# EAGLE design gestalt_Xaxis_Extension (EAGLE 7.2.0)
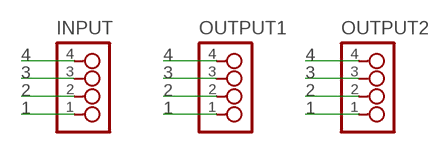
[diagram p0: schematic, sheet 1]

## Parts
INPUT  4_PIN_HEADERHEADER  [SMT_PINS_4]
OUTPUT1  4_PIN_HEADERHEADER  [SMT_PINS_4]
OUTPUT2  4_PIN_HEADERHEADER  [SMT_PINS_4]

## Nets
1: INPUT.1 OUTPUT1.1 OUTPUT2.1
2: INPUT.2 OUTPUT1.2 OUTPUT2.2
3: INPUT.3 OUTPUT1.3 OUTPUT2.3
4: INPUT.4 OUTPUT1.4 OUTPUT2.4

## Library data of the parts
INPUT OUTPUT1 OUTPUT2 = ng:4_PIN_HEADER: 4 SMT pin pads

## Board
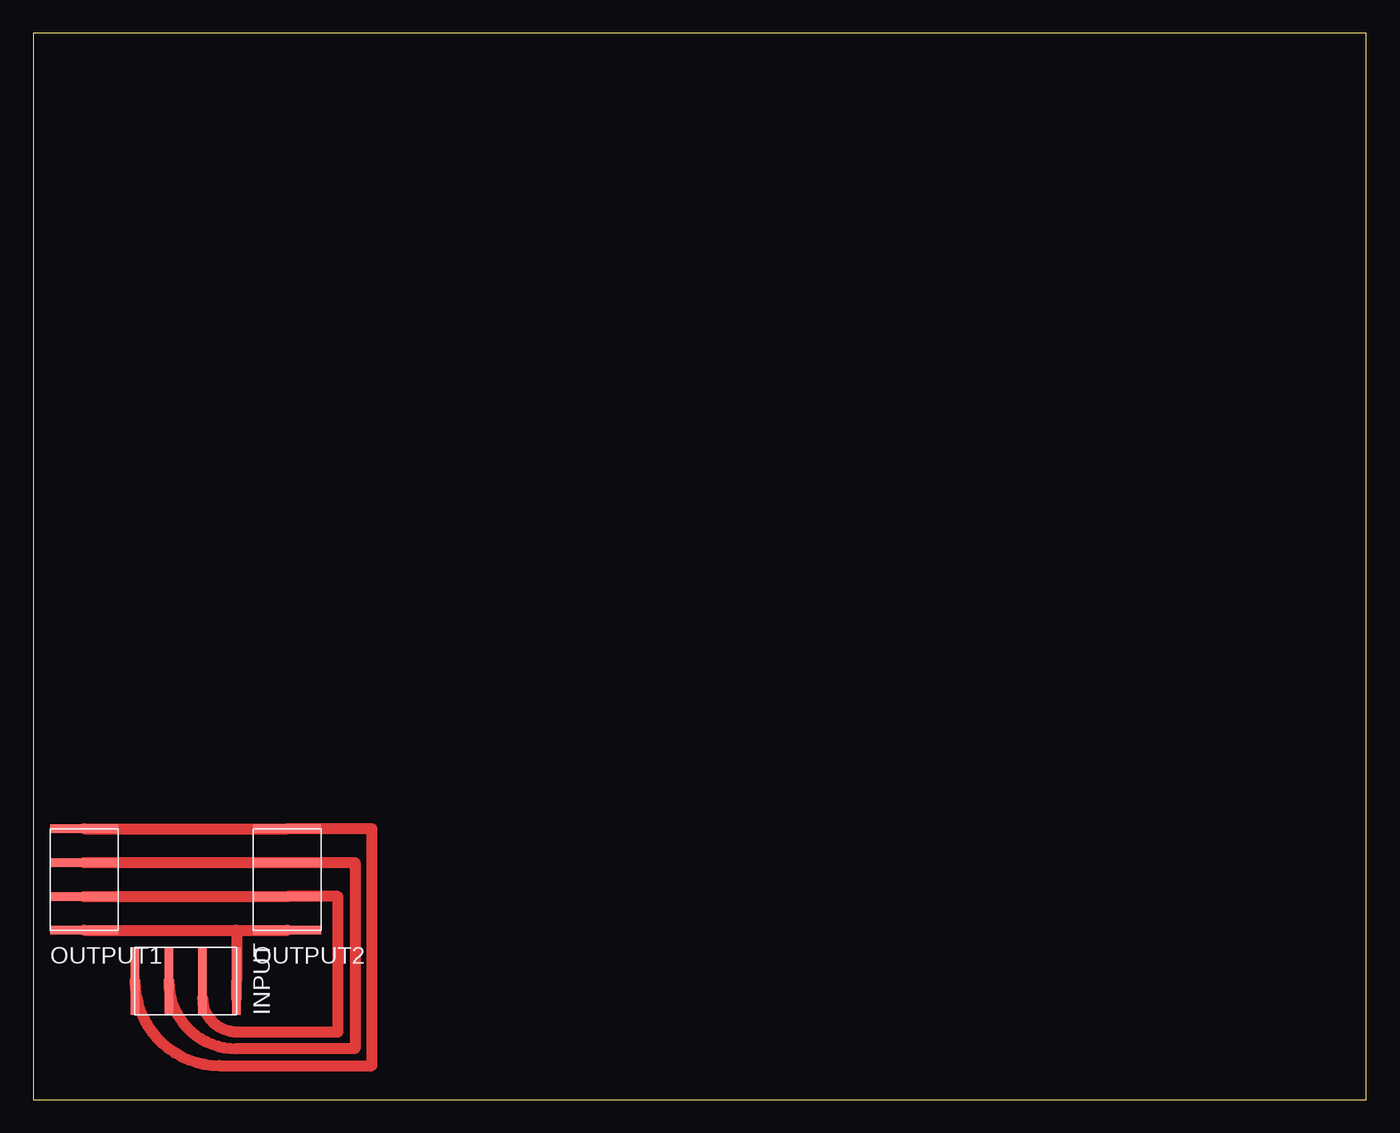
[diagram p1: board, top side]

Size 100 x 80 mm. Coordinates in mm from the lower left corner, seen from the top.
Outline: 0,0 100,0 100,80 0,80 0,0
Copper layers (1*16): Top 0.035mm / dielectric 1.5mm / Bottom 0.035mm
Design rules "default *": minimum track width 10mil, minimum drill 24mil, track to track 0.4mm, track to pad 0.4mm, pad to pad 0.4mm, via to via 0.4mm, smd to smd 8mil, copper to edge 40mil, drill to drill 8mil, minimum pad ring 10mil, minimum via ring 8mil, stop-mask expansion 4mil, vias tented up to drill 0mil, thermal gap 10mil

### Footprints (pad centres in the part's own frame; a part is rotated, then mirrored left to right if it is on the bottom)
SMT_PINS_4 = smd 5.08 x 0.635: 1 0,0; 2 0,2.54; 3 0,5.08; 4 0,7.62

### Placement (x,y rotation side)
INPUT  15.24,8.89 90 top
OUTPUT1  3.81,12.7 0 top
OUTPUT2  19.05,12.7 0 top

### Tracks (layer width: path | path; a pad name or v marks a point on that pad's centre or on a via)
1
  Top 0.813: OUTPUT1.1 15.24,12.7 | 15.24,12.7 OUTPUT2.1 | 15.24,12.7 INPUT.1 15.24,7.62
2
  Top 0.406: INPUT.2 12.7,7.62
  Top 0.813: OUTPUT1.2 OUTPUT2.2 22.86,15.24 22.86,5.08 15.24,5.08 arc-90 12.7,7.62
3
  Top 0.813: OUTPUT1.3 OUTPUT2.3 24.13,17.78 24.13,3.81 15.24,3.81 arc-90 INPUT.3
4
  Top 0.813: OUTPUT1.4 OUTPUT2.4 25.4,20.32 25.4,2.54 13.97,2.54 arc-90 INPUT.4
